|   IBIS model for TI AM261
[IBIS Ver]   5.1
[Disclaimer]   Please be aware that in the absence of a written agreement
|   Texas Instruments(TI) assumes no liability for:
|   (1) The accuracy of the IBIS models provided to your company,
|   however, the IBIS model is compliant to industry standard
|   IQ Level 2a.  Refer to IBIS Quality Section below for
|   for full details.
|   (2) The proper functioning of these Models in your design
|   or for any resulting applications
|   (3) Infringement of patents, copyrights or intellectual
|   property rights resulting from your use of these
|   models.
|   TI provides IBIS Models as a service to our customers and
|   therefore reserves the right to limit distribution of the
|   Models.  The information is subject to change without notice.
[File Name]  zej.ibs
[File Rev]   0.1
|   -Initial version
|   -Updated Package model
[Date]   10 October 2024
[Source]   Texas Instruments Incorporated
[Copyright]   Property of Texas Instruments Incorporated.
|   Unauthorized reproduction and/or distribution is strictly.
|   prohibited.
|   This product is protected under copyright law and trade
|   secret law as an unpublished work.
|   Created 2012,(C) Copyright 1999-2012,
|   Texas Instruments Incorporated., All Rights Reserved.
|   These commodities are under the U.S. Government
|   distribution license control. As such,they are not to be
|   re-exported without the prior approval of the U.S.
|   Department of Commerce.
[Notes]
   ADC pins are marked as NC
   USB pins are marked as NC
   Clock pins are marked as NC
   nReset pin marked as NC
|   Revision History
|   GERNERAL COMMENT: All IBIS Quality Notes below reflect latest release
|   and version of IBIS File
|   File passes ibischk6.0 with 0 errors and 35 warnings
|   Component AM261
[Component] AM261
[Manufacturer] TEXAS INSTRUMENTS
[Package Model] AM261_ZEJ
[Package]
|   typ   min   max
R_pkg   0.17037   0.058312   0.31733
L_pkg   2.972e-9   9.974e-10   4.815e-9
C_pkg   4.94e-13   3.685e-13   7.579e-13
[Pin]   Signal_name   model_name
E11   VDD   POWER
F12   VDD   POWER
H12   VDD   POWER
K12   VDD   POWER
M12   VDD   POWER
E5   VDD   POWER
E7   VDD   POWER
E9   VDD   POWER
G5   VDD   POWER
J5   VDD   POWER
L5   VDD   POWER
M6   VDD   POWER
N9   VDDA18_LDO   POWER
N6   VDDA18_OSC_PLL   POWER
N4   VDDA18_USB   POWER
M10   VDDA33   POWER
M8   VDDA33   POWER
M4   VDDA33_USB   POWER
D10   VDDAR2   POWER
G4   VDDAR3   POWER
D6   VDDS18   POWER
D12   VDDS18   POWER
G13   VDDS18   POWER
K13   VDDS18   POWER
K4   VDDS18   POWER
E4   VDDS18   POWER
N13   VDDS18   POWER
D9   VDDS18   POWER
P4   VDDS18_LDO   POWER
D4   VDDSHV_A   POWER
D7   VDDSHV_A   POWER
D11   VDDSHV_A   POWER
F13   VDDSHV_A   POWER
J13   VDDSHV_A   POWER
L4   VDDSHV_B   POWER
N12   VDDSHV_C   POWER
J4   VDDSHV_D   POWER
H4   VDDSHV_D   POWER
M13   VDDSHV_E   POWER
N5   VDDSHV_F   POWER
N8   VDD_TEMP   NC
P11   ADC0_AIN0   NC
N11   ADC0_AIN1   NC
R11   ADC0_AIN2   NC
P12   ADC0_AIN3   NC
T12   ADC0_AIN4   NC
R12   ADC0_AIN5   NC
T13   ADC0_AIN6   NC
R10   ADC1_AIN0   NC
N10   ADC1_AIN1   NC
P10   ADC1_AIN2   NC
P9   ADC1_AIN3   NC
T9   ADC1_AIN4   NC
R9   ADC1_AIN5   NC
R8   ADC1_AIN6   NC
R7   ADC2_AIN0   NC
P7   ADC2_AIN1   NC
P8   ADC2_AIN2   NC
P6   ADC2_AIN3   NC
R6   ADC2_AIN4   NC
N7   ADC2_AIN5   NC
T6   ADC2_AIN6   NC
R13   ADC_CAL0   NC
T10   ADC_VREFHI_G0   NC
T7   ADC_VREFHI_G1   NC
T11   ADC_VREFLO_G0   NC
T8   ADC_VREFLO_G1   NC
T4   ATESTV1   NC
T5   DAC_OUT   NC
P13   DAC_VREF0   NC
N3   GPIO0   bc1833dv40dcpbfbp18ll_rxll_ssdlv
M3   GPIO1   bc1833dv40dcpbfbp18ll_rxll_ssdlv
L2   GPIO2   bc1833dv40dcpbfbp18ll_rxll_ssdlv
M2   GPIO3   bc1833dv40dcpbfbp18ll_ssdlv
N1   GPIO4   bc1833dv40dcpbfbp18ll_ssdlv
L3   GPIO5   bc1833dv40dcpbfbp18ll_rxll_ssdlv
N2   GPIO6   bc1833dv40dcpbfbp18ll_rxll_ssdlv
J3   GPIO7   bc1833dv40dcpbfbp18ll_rxll_ssdlv
K1   GPIO8   bc1833dv40dcpbfbp18ll_rxll_ssdlv
K2   GPIO9   bc1833dv40dcpbfbp18ll_rxll_ssdlv
J2   GPIO10   bc1833dv40dcpbfbp18ll_rxll_ssdlv
B11   GPIO11   bc1833dv40dcpbfbp18ll_rxll_ssdlh
A12   GPIO12   bc1833dv40dcpbfbp18ll_ssdlh
A10   GPIO13   bc1833dv40dcpbfbp18ll_ssdlh
A11   GPIO14   bc1833dv40dcpbfbp18ll_rxll_ssdlh
B9   GPIO15   bc1833dv40dcpbfbp18ll_rxll_ssdlh
B10   GPIO16   bc1833dv40dcpbfbp18ll_rxll_ssdlh
A9   GPIO17   bc1833dv40dcpbfbp18ll_rxll_ssdlh
C11   GPIO18   bc1833dv40dcpbfbp18ll_rxll_ssdlh
C10   GPIO19   bc1833dv40dcpbfbp18ll_rxll_ssdlh
D8   GPIO20   bc1833dv40dcpbfbp18ll_rxll_ssdlh
B8   GPIO21   bc1833dv40dcpbfbp18ll_rxll_ssdlh
C9   GPIO22   bc1833dv40dcpbfbp18ll_rxll_ssdlh
B7   GPIO23   bc1833dv40dcpbfbp18ll_rxll_ssdlh
A8   GPIO24   bc1833dv40dcpbfbp18ll_rxll_ssdlh
C8   GPIO25   bc1833dv40dcpbfbp18ll_rxll_ssdlh
A7   GPIO26   bc1833dv40dcpbfbp18ll_rxll_ssdlh
A6   GPIO27   bc1833dv40dcpbfbp18ll_rxll_ssdlh
B6   GPIO28   bc1833dv40dcpbfbp18ll_rxll_ssdlh
P16   GPIO29   bc1833dv40dcpbfbp18ll_rxll_ssdlv_135u
M14   GPIO30   bc1833dv40dcpbfbp18ll_rxll_ssdlv_135u
P14   GPIO31   bc1833dv40dcpbfbp18ll_rxll_ssdlh
P15   GPIO32   bc1833dv40dcpbfbp18ll_rxll_ssdlh
R16   GPIO33   bc1833dv40dcpbfbp18ll_rxll_ssdlh
N14   GPIO34   bc1833dv40dcpbfbp18ll_rxll_ssdlv_135u
L15   GPIO35   bc1833dv40dcpbfbp18ll_rxll_ssdlv_135u
M16   GPIO36   bc1833dv40dcpbfbp18ll_rxll_ssdlv_135u
N15   GPIO37   bc1833dv40dcpbfbp18ll_rxll_ssdlv_135u
N16   GPIO38   bc1833dv40dcpbfbp18ll_rxll_ssdlv_135u
L13   GPIO39   bc1833dv40dcpbfbp18ll_rxll_ssdlv_135u
M15   GPIO40   bc1833dv40dcpbfbp18ll_rxll_ssdlv_135u
L16   GPIO41   bc1833dv40dcpbfbp18ll_rxll_ssdlv_135u
L14   GPIO42   bc1833dv40dcpbfbp18ll_rxll_ssdlv_135u
A4   GPIO43   bc1833dv40dcpbfbp18ll_rxll_ssdlh_135u
A5   GPIO44   bc1833dv40dcpbfbp18ll_rxll_ssdlh_135u
B4   GPIO45   bc1833dv40dcpbfbp18ll_rxll_ssdlh_135u
C5   GPIO46   bc1833dv40dcpbfbp18ll_rxll_ssdlh_135u
A3   GPIO47   bc1833dv40dcpbfbp18ll_rxll_ssdlh_135u
A2   GPIO48   bc1833dv40dcpbfbp18ll_rxll_ssdlh_135u
B2   GPIO49   bc1833dv40dcpbfbp18ll_rxll_ssdlh_135u
C4   GPIO50   bc1833dv40dcpbfbp18ll_rxll_ssdlv
B1   GPIO51   bc1833dv40dcpbfbp18ll_rxll_ssdlv
C1   GPIO52   bc1833dv40dcpbfbp18ll_rxll_ssdlv
C2   GPIO53   bc1833dv40dcpbfbp18ll_rxll_ssdlv
D3   GPIO54   bc1833dv40dcpbfbp18ll_rxll_ssdlv
E3   GPIO55   bc1833dv40dcpbfbp18ll_rxll_ssdlv
F4   GPIO56   bc1833dv40dcpbfbp18ll_rxll_ssdlv
D2   GPIO57   bc1833dv40dcpbfbp18ll_rxll_ssdlv
D1   GPIO58   bc1833dv40dcpbfbp18ll_rxll_ssdlv
E2   GPIO59   bc1833dv40dcpbfbp18ll_rxll_ssdlv
E1   GPIO60   bc1833dv40dcpbfbp18ll_rxll_ssdlv
F2   GPIO61   bc1833dv40dcpbfbp18ll_rxll_ssdlv
F3   GPIO62   bc1833dv40dcpbfbp18ll_rxll_ssdlv
G3   GPIO66   bc1833dv40dcpbfbp18ll_rxll_ssdlv
G2   GPIO67   bc1833dv40dcpbfbp18ll_rxll_ssdlv
H3   GPIO68   bc1833dv40dcpbfbp18ll_rxll_ssdlv
H2   GPIO69   bc1833dv40dcpbfbp18ll_rxll_ssdlv
G1   GPIO70   bc1833dv40dcpbfbp18ll_rxll_ssdlv
R14   GPIO71   bc1833dv40dcpbfbp18ll_rxll_ssdlh
T14   GPIO72   bc1833dv40dcpbfbp18ll_rxll_ssdlh
T15   GPIO73   bc1833dv40dcpbfbp18ll_rxll_ssdlh
R15   GPIO74   bc1833dv40dcpbfbp18ll_rxll_ssdlh
M1   GPIO75   bc1833dv40dcpbfbp18ll_rxll_ssdlv
L1   GPIO76   bc1833dv40dcpbfbp18ll_rxll_ssdlv
K15   GPIO85   bc1833dv40dcpbfbp18ll_rxll_ssdlv_135u
K16   GPIO86   bc1833dv40dcpbfbp18ll_rxll_ssdlv_135u
F14   GPIO87   bc1833dv40dcpbfbp18ll_rxll_ssdlv_135u
E15   GPIO88   bc1833dv40dcpbfbp18ll_rxll_ssdlv_135u
E16   GPIO89   bc1833dv40dcpbfbp18ll_rxll_ssdlv_135u
E14   GPIO90   bc1833dv40dcpbfbp18ll_rxll_ssdlv_135u
H15   GPIO91   bc1833dv40dcpbfbp18ll_rxll_ssdlv_135u
G15   GPIO92   bc1833dv40dcpbfbp18ll_rxll_ssdlv_135u
K14   GPIO93   bc1833dv40dcpbfbp18ll_rxll_ssdlv_135u
H14   GPIO94   bc1833dv40dcpbfbp18ll_rxll_ssdlv_135u
G16   GPIO95   bc1833dv40dcpbfbp18ll_rxll_ssdlv_135u
J14   GPIO96   bc1833dv40dcpbfbp18ll_rxll_ssdlv_135u
F16   GPIO97   bc1833dv40dcpbfbp18ll_rxll_ssdlv_135u
H16   GPIO98   bc1833dv40dcpbfbp18ll_rxll_ssdlv_135u
J15   GPIO99   bc1833dv40dcpbfbp18ll_rxll_ssdlv_135u
J16   GPIO100   bc1833dv40dcpbfbp18ll_rxll_ssdlv_135u
F15   GPIO101   bc1833dv40dcpbfbp18ll_rxll_ssdlv_135u
G14   GPIO102   bc1833dv40dcpbfbp18ll_rxll_ssdlv_135u
E13   GPIO107   bc1833dv40dcpbfbp18ll_rxll_ssdlv_135u
D15   GPIO108   bc1833dv40dcpbfbp18ll_rxll_ssdlv_135u
D14   GPIO109   bc1833dv40dcpbfbp18ll_rxll_ssdlv_135u
D16   GPIO110   bc1833dv40dcpbfbp18ll_rxll_ssdlv_135u
P3   GPIO121   bc1833dv40dcpbfbp18ll_rxll_ssdlh
C15   GPIO122   bc1833dv40dcpbfbp18ll_rxll_ssdlh
A15   GPIO123   bc1833dv40dcpbfbp18ll_rxll_ssdlh
C16   GPIO124   bc1833dv40dcpbfbp18ll_rxll_ssdlh
C14   GPIO125   bc1833dv40dcpbfbp18ll_rxll_ssdlh
B16   GPIO126   bc1833dv40dcpbfbp18ll_rxll_ssdlh
A14   GPIO127   bc1833dv40dcpbfbp18ll_rxll_ssdlh
B15   GPIO128   bc1833dv40dcpbfbp18ll_rxll_ssdlh
B14   GPIO129   bc1833dv40dcpbfbp18ll_rxll_ssdlh
D13   GPIO130   bc1833dv40dcpbfbp18ll_rxll_ssdlh
C13   GPIO131   bc1833dv40dcpbfbp18ll_rxll_ssdlh
C12   GPIO132   bc1833dv40dcpbfbp18ll_rxll_ssdlh
B13   GPIO133   bc1833dv40dcpbfbp18ll_rxll_ssdlh
B12   GPIO134   bi2c1833dvfzp18_ssdlh
A13   GPIO135   bi2c1833dvfzp18_ssdlh
H1   GPIO138   bc1833dv40dcpbfbp18ll_rxll_ssdlv
R1   GPIO139   NC
P1   GPIO140   NC
P2   PORZ   ihhv1833dvhyp18ll_ssdhv
B3   SAFETY_ERRORN   bc1833dv40dcpbfbp18ll_ssdlh_135u
C6   TCK   iq1833dvtckpbfbp18ll_ssdhh_135u
D5   TDI   bc1833dv40dcpbfbp18ll_ssdlh_135u
B5   TDO   bc1833dv40dcpbfbp18ll_ssdlh_135u
P5   TEMPCAL   NC
C7   TMS   bc1833dv40dcpbfbp18ll_ssdlh_135u
H13   VNWA   POWER
K3   VPP   POWER
R5   VSYS_MON   NC
C3   WARMRSTN   bc1833dv40dcpbfbp18ll_od_fs_cmphdl_ssdlv
T3   XTAL_XI   NC
T2   XTAL_XO   NC
A1   VSS   GND
A16   VSS   GND
F5   VSS   GND
E6   VSS   GND
E8   VSS   GND
E10   VSS   GND
E12   VSS   GND
G6   VSS   GND
F6   VSS   GND
G7   VSS   GND
F7   VSS   GND
G8   VSS   GND
F8   VSS   GND
G9   VSS   GND
F9   VSS   GND
G10   VSS   GND
F10   VSS   GND
G11   VSS   GND
F11   VSS   GND
H6   VSS   GND
H7   VSS   GND
H8   VSS   GND
H9   VSS   GND
H10   VSS   GND
H11   VSS   GND
K5   VSS   GND
K6   VSS   GND
J6   VSS   GND
K7   VSS   GND
J7   VSS   GND
K8   VSS   GND
J8   VSS   GND
K9   VSS   GND
J9   VSS   GND
K10   VSS   GND
J10   VSS   GND
K11   VSS   GND
J11   VSS   GND
L6   VSS   GND
L7   VSS   GND
L8   VSS   GND
L9   VSS   GND
L10   VSS   GND
L11   VSS   GND
M5   VSS   GND
M7   VSS   GND
G12   VSS   GND
H5   VSS   GND
J12   VSS   GND
L12   VSS   GND
R2   VSS   GND
T1   VSS   GND
R3   VSS   GND
R4   VSS   GND
T16   VSS   GND
M9   VSSA   GND
M11   VSSA   GND
|   BC1833DV40DCPBFBP18LL_SSDLH
[Model Selector] bc1833dv40dcpbfbp18ll_ssdlh
|SC1 IS A SLEW RATE CONTROL PIN
|5% SUPPLY VARIATION MODES WITH 1.8V NOM SUPPLY
BC40D_H_PUPDOFF_5P_SC1_1P8  Cell operated at 1.8(nom)
|BC40D_H_PUPDOFF_5P_SC1_1P8; BUFFER WITH WEAK PULUP/PULLDOWN OFF AT 5% SUPPLY
|VARIATION WITH SC1=1 MEANING SLOW MODE OF OPERATION
BC40D_H_PD_ON_5P_!SC1_1P8  Cell operated at 1.8(nom)
|BC40D_H_PD_ON_5P_!SC1_1P8; BUFFER WITH WEAK_PULLDOWN_ON AT 5% SUPPLY
|VARIATION WITH SC1=0 MEANING FAST MODE OF OPERATION
BC40D_H_PD_ON_5P_SC1_1P8  Cell operated at 1.8(nom)
|BC40D_H_PD_ON_5P_SC1_1P8; BUFFER WITH WEAK_PULLDOWN_ON AT 5% SUPPLY
|VARIATION WITH SC1=1 MEANING SLOW MODE OF OPERATION
BC40D_H_PU_ON_5P_!SC1_1P8  Cell operated at 1.8(nom)
|BC40D_H_PU_ON_5P_!SC1_1P8; BUFFER WITH WEAK_PULLUP_ON AT 5% SUPPLY
|VARIATION WITH SC1=0 MEANING FAST MODE OF OPERATION
BC40D_H_PUPDOFF_5P_!SC1_1P8  Cell operated at 1.8(nom)
|BC40D_H_PUPDOFF_5P_!SC1_1P8; BUFFER WITH WEAK PULUP/PULLDOWN OFF AT 5% SUPPLY
|VARIATION WITH SC1=0 MEANING FAST MODE OF OPERATION
BC40D_H_PU_ON_5P_SC1_1P8  Cell operated at 1.8(nom)
|BC40D_H_PU_ON_5P_SC1_1P8; BUFFER WITH WEAK_PULLUP_ON AT 5% SUPPLY
|VARIATION WITH SC1=1 MEANING SLOW MODE OF OPERATION
|5% SUPPLY VARIATION MODES WITH 3.3V NOM SUPPLY
BC40D_H_PUPDOFF_5P_SC1_3P3  Cell operated at 3.3(nom)
|BC40D_H_PUPDOFF_5P_SC1_3P3; BUFFER WITH WEAK PULUP/PULLDOWN OFF AT 5% SUPPLY
|VARIATION WITH SC1=1 MEANING SLOW MODE OF OPERATION
BC40D_H_PD_ON_5P_!SC1_3P3  Cell operated at 3.3(nom)
|BC40D_H_PD_ON_5P_!SC1_3P3; BUFFER WITH WEAK_PULLDOWN_ON AT 5% SUPPLY
|VARIATION WITH SC1=0 MEANING FAST MODE OF OPERATION
BC40D_H_PD_ON_5P_SC1_3P3  Cell operated at 3.3(nom)
|BC40D_H_PD_ON_5P_SC1_3P3; BUFFER WITH WEAK_PULLDOWN_ON AT 5% SUPPLY
|VARIATION WITH SC1=1 MEANING SLOW MODE OF OPERATION
BC40D_H_PU_ON_5P_!SC1_3P3  Cell operated at 3.3(nom)
|BC40D_H_PU_ON_5P_!SC1_3P3; BUFFER WITH WEAK_PULLUP_ON AT 5% SUPPLY
|VARIATION WITH SC1=0 MEANING FAST MODE OF OPERATION
BC40D_H_PUPDOFF_5P_!SC1_3P3  Cell operated at 3.3(nom)
|BC40D_H_PUPDOFF_5P_!SC1_3P3; BUFFER WITH WEAK PULUP/PULLDOWN OFF AT 5% SUPPLY
|VARIATION WITH SC1=0 MEANING FAST MODE OF OPERATION
BC40D_H_PU_ON_5P_SC1_3P3  Cell operated at 3.3(nom)
|BC40D_H_PU_ON_5P_SC1_3P3; BUFFER WITH WEAK_PULLUP_ON AT 5% SUPPLY
|VARIATION WITH SC1=1 MEANING SLOW MODE OF OPERATION
| 10% SUPPLY VARIATION MODES WITH 1.8V NOM SUPPLY
BC40D_H_PUPDOFF_10P_SC1_1P8  Cell operated at 1.8(nom)
|BC40D_H_PUPDOFF_10P_SC1_1P8; BUFFER WITH WEAK PULUP/PULLDOWN OFF AT 10% SUPPLY
|VARIATION WITH SC1=1 MEANING SLOW MODE OF OPERATION
BC40D_H_PD_ON_10P_!SC1_1P8  Cell operated at 1.8(nom)
|BC40D_H_PD_ON_10P_!SC1_1P8; BUFFER WITH WEAK_PULLDOWN_ON AT 10% SUPPLY
|VARIATION WITH SC1=0 MEANING FAST MODE OF OPERATION
BC40D_H_PD_ON_10P_SC1_1P8  Cell operated at 1.8(nom)
|BC40D_H_PD_ON_10P_SC1_1P8; BUFFER WITH WEAK_PULLDOWN_ON AT 10% SUPPLY
|VARIATION WITH SC1=1 MEANING SLOW MODE OF OPERATION
BC40D_H_PU_ON_10P_!SC1_1P8  Cell operated at 1.8(nom)
|BC40D_H_PU_ON_10P_!SC1_1P8; BUFFER WITH WEAK_PULLUP_ON AT 10% SUPPLY
|VARIATION WITH SC1=0 MEANING FAST MODE OF OPERATION
BC40D_H_PUPDOFF_10P_!SC1_1P8  Cell operated at 1.8(nom)
|BC40D_H_PUPDOFF_10P_!SC1_1P8; BUFFER WITH WEAK PULUP/PULLDOWN OFF AT 10% SUPPLY
|VARIATION WITH SC1=0 MEANING FAST MODE OF OPERATION
BC40D_H_PU_ON_10P_SC1_1P8  Cell operated at 1.8(nom)
|BC40D_H_PU_ON_10P_SC1_1P8; BUFFER WITH WEAK_PULLUP_ON AT 10% SUPPLY
|VARIATION WITH SC1=1 MEANING SLOW MODE OF OPERATION
| 10% SUPPLY VARIATION MODES WITH 3.3V NOM SUPPLY
BC40D_H_PUPDOFF_10P_SC1_3P3  Cell operated at 3.3(nom)
|BC40D_H_PUPDOFF_10P_SC1_3P3; BUFFER WITH WEAK PULUP/PULLDOWN OFF AT 10% SUPPLY
|VARIATION WITH SC1=1 MEANING SLOW MODE OF OPERATION
BC40D_H_PD_ON_10P_!SC1_3P3  Cell operated at 3.3(nom)
|BC40D_H_PD_ON_10P_!SC1_3P3; BUFFER WITH WEAK_PULLDOWN_ON 10% SUPPLY
|VARIATION WITH SC1=0 MEANING FAST MODE OF OPERATION
BC40D_H_PD_ON_10P_SC1_3P3  Cell operated at 3.3(nom)
|BC40D_H_PD_ON_10P_SC1_3P3; BUFFER WITH WEAK_PULLDOWN_ON AT 10% SUPPLY
|VARIATION WITH SC1=1 MEANING SLOW MODE OF OPERATION
BC40D_H_PU_ON_10P_!SC1_3P3  Cell operated at 3.3(nom)
|BC40D_H_PU_ON_10P_!SC1_3P3; BUFFER WITH WEAK_PULLUP_ON AT 10% SUPPLY
|VARIATION WITH SC1=0 MEANING FAST MODE OF OPERATION
BC40D_H_PUPDOFF_10P_!SC1_3P3  Cell operated at 3.3(nom)
|BC40D_H_PUPDOFF_10P_!SC1_3P3; BUFFER WITH WEAK PULUP/PULLDOWN OFF AT 10% SUPPLY
|VARIATION WITH SC1=0 MEANING FAST MODE OF OPERATION
BC40D_H_PU_ON_10P_SC1_3P3  Cell operated at 3.3(nom)
|BC40D_H_PU_ON_10P_SC1_3P3; BUFFER WITH WEAK_PULLUP_ON AT 10% SUPPLY
|VARIATION WITH SC1=1 MEANING SLOW MODE OF OPERATION
|   BC1833DV40DCPBFBP18LL_SSDLV
[Model Selector] bc1833dv40dcpbfbp18ll_ssdlv
|SC1 IS A SLEW RATE CONTROL PIN
|5% SUPPLY VARIATION MODES WITH 1.8V NOM SUPPLY
BC40D_V_PUPDOFF_5P_SC1_1P8  Cell operated at 1.8(nom)
|BC40D_V_PUPDOFF_5P_SC1_1P8; BUFFER WITH WEAK PULUP/PULLDOWN OFF AT 5% SUPPLY
|VARIATION WITH SC1=1 MEANING SLOW MODE OF OPERATION
BC40D_V_PD_ON_5P_!SC1_1P8  Cell operated at 1.8(nom)
|BC40D_V_PD_ON_5P_!SC1_1P8; BUFFER WITH WEAK_PULLDOWN_ON AT 5% SUPPLY
|VARIATION WITH SC1=0 MEANING FAST MODE OF OPERATION
BC40D_V_PD_ON_5P_SC1_1P8  Cell operated at 1.8(nom)
|BC40D_V_PD_ON_5P_SC1_1P8; BUFFER WITH WEAK_PULLDOWN_ON AT 5% SUPPLY
|VARIATION WITH SC1=1 MEANING SLOW MODE OF OPERATION
BC40D_V_PU_ON_5P_!SC1_1P8  Cell operated at 1.8(nom)
|BC40D_V_PU_ON_5P_!SC1_1P8; BUFFER WITH WEAK_PULLUP_ON AT 5% SUPPLY
|VARIATION WITH SC1=0 MEANING FAST MODE OF OPERATION
BC40D_V_PUPDOFF_5P_!SC1_1P8  Cell operated at 1.8(nom)
|BC40D_V_PUPDOFF_5P_!SC1_1P8; BUFFER WITH WEAK PULUP/PULLDOWN OFF AT 5% SUPPLY
|VARIATION WITH SC1=0 MEANING FAST MODE OF OPERATION
BC40D_V_PU_ON_5P_SC1_1P8  Cell operated at 1.8(nom)
|BC40D_V_PU_ON_5P_SC1_1P8; BUFFER WITH WEAK_PULLUP_ON AT 5% SUPPLY
|VARIATION WITH SC1=1 MEANING SLOW MODE OF OPERATION
|5% SUPPLY VARIATION MODES WITH 3.3V NOM SUPPLY
BC40D_V_PUPDOFF_5P_SC1_3P3  Cell operated at 3.3(nom)
|BC40D_V_PUPDOFF_5P_SC1_3P3; BUFFER WITH WEAK PULUP/PULLDOWN OFF AT 5% SUPPLY
|VARIATION WITH SC1=1 MEANING SLOW MODE OF OPERATION
BC40D_V_PD_ON_5P_!SC1_3P3  Cell operated at 3.3(nom)
|BC40D_V_PD_ON_5P_!SC1_3P3; BUFFER WITH WEAK_PULLDOWN_ON AT 5% SUPPLY
|VARIATION WITH SC1=0 MEANING FAST MODE OF OPERATION
BC40D_V_PD_ON_5P_SC1_3P3  Cell operated at 3.3(nom)
|BC40D_V_PD_ON_5P_SC1_3P3; BUFFER WITH WEAK_PULLDOWN_ON AT 5% SUPPLY
|VARIATION WITH SC1=1 MEANING SLOW MODE OF OPERATION
BC40D_V_PU_ON_5P_!SC1_3P3  Cell operated at 3.3(nom)
|BC40D_V_PU_ON_5P_!SC1_3P3; BUFFER WITH WEAK_PULLUP_ON AT 5% SUPPLY
|VARIATION WITH SC1=0 MEANING FAST MODE OF OPERATION
BC40D_V_PUPDOFF_5P_!SC1_3P3  Cell operated at 3.3(nom)
|BC40D_V_PUPDOFF_5P_!SC1_3P3; BUFFER WITH WEAK PULUP/PULLDOWN OFF AT 5% SUPPLY
|VARIATION WITH SC1=0 MEANING FAST MODE OF OPERATION
BC40D_V_PU_ON_5P_SC1_3P3  Cell operated at 3.3(nom)
|BC40D_V_PU_ON_5P_SC1_3P3; BUFFER WITH WEAK_PULLUP_ON AT 5% SUPPLY
|VARIATION WITH SC1=1 MEANING SLOW MODE OF OPERATION
| 10% SUPPLY VARIATION MODES WITH 1.8V NOM SUPPLY
BC40D_V_PUPDOFF_10P_SC1_1P8  Cell operated at 1.8(nom)
|BC40D_V_PUPDOFF_10P_SC1_1P8; BUFFER WITH WEAK PULUP/PULLDOWN OFF AT 10% SUPPLY
|VARIATION WITH SC1=1 MEANING SLOW MODE OF OPERATION
BC40D_V_PD_ON_10P_!SC1_1P8  Cell operated at 1.8(nom)
|BC40D_V_PD_ON_10P_!SC1_1P8; BUFFER WITH WEAK_PULLDOWN_ON AT 10% SUPPLY
|VARIATION WITH SC1=0 MEANING FAST MODE OF OPERATION
BC40D_V_PD_ON_10P_SC1_1P8  Cell operated at 1.8(nom)
|BC40D_V_PD_ON_10P_SC1_1P8; BUFFER WITH WEAK_PULLDOWN_ON AT 10% SUPPLY
|VARIATION WITH SC1=1 MEANING SLOW MODE OF OPERATION
BC40D_V_PU_ON_10P_!SC1_1P8  Cell operated at 1.8(nom)
|BC40D_V_PU_ON_10P_!SC1_1P8; BUFFER WITH WEAK_PULLUP_ON AT 10% SUPPLY
|VARIATION WITH SC1=0 MEANING FAST MODE OF OPERATION
BC40D_V_PUPDOFF_10P_!SC1_1P8  Cell operated at 1.8(nom)
|BC40D_V_PUPDOFF_10P_!SC1_1P8; BUFFER WITH WEAK PULUP/PULLDOWN OFF AT 10% SUPPLY
|VARIATION WITH SC1=0 MEANING FAST MODE OF OPERATION
BC40D_V_PU_ON_10P_SC1_1P8  Cell operated at 1.8(nom)
|BC40D_V_PU_ON_10P_SC1_1P8; BUFFER WITH WEAK_PULLUP_ON AT 10% SUPPLY
|VARIATION WITH SC1=1 MEANING SLOW MODE OF OPERATION
| 10% SUPPLY VARIATION MODES WITH 3.3V NOM SUPPLY
BC40D_V_PUPDOFF_10P_SC1_3P3  Cell operated at 3.3(nom)
|BC40D_V_PUPDOFF_10P_SC1_3P3; BUFFER WITH WEAK PULUP/PULLDOWN OFF AT 10% SUPPLY
|VARIATION WITH SC1=1 MEANING SLOW MODE OF OPERATION
BC40D_V_PD_ON_10P_!SC1_3P3  Cell operated at 3.3(nom)
|BC40D_V_PD_ON_10P_!SC1_3P3; BUFFER WITH WEAK_PULLDOWN_ON 10% SUPPLY
|VARIATION WITH SC1=0 MEANING FAST MODE OF OPERATION
BC40D_V_PD_ON_10P_SC1_3P3  Cell operated at 3.3(nom)
|BC40D_V_PD_ON_10P_SC1_3P3; BUFFER WITH WEAK_PULLDOWN_ON AT 10% SUPPLY
|VARIATION WITH SC1=1 MEANING SLOW MODE OF OPERATION
BC40D_V_PU_ON_10P_!SC1_3P3  Cell operated at 3.3(nom)
|BC40D_V_PU_ON_10P_!SC1_3P3; BUFFER WITH WEAK_PULLUP_ON AT 10% SUPPLY
|VARIATION WITH SC1=0 MEANING FAST MODE OF OPERATION
BC40D_V_PUPDOFF_10P_!SC1_3P3  Cell operated at 3.3(nom)
|BC40D_V_PUPDOFF_10P_!SC1_3P3; BUFFER WITH WEAK PULUP/PULLDOWN OFF AT 10% SUPPLY
|VARIATION WITH SC1=0 MEANING FAST MODE OF OPERATION
BC40D_V_PU_ON_10P_SC1_3P3  Cell operated at 3.3(nom)
|BC40D_V_PU_ON_10P_SC1_3P3; BUFFER WITH WEAK_PULLUP_ON AT 10% SUPPLY
|VARIATION WITH SC1=1 MEANING SLOW MODE OF OPERATION
|   BI2C1833DVFZP18_SSDLH
[Model Selector] bi2c1833dvfzp18_ssdlh
BI2C1833_NORAML_5P_1P8  Cell operated at 1.8(nom)
|BI2C1833_NORAML_5P_1P8; I2C MODE AT 1.8V WITH 5% SUPPLY VARIATION
BI2C1833_NORAML_5P_3P3  Cell operated at 3.3(nom)
|BI2C1833_NORAML_5P_3P3; I2C MODE AT 3.3V WITH 5% SUPPLY VARIATION
BI2C1833_NORAML_10P_1P8  Cell operated at 1.8(nom)
|BI2C1833_NORAML_10P_1P8; I2C MODE AT 1.8V WITH 10% SUPPLY VARIATION
BI2C1833_NORAML_10P_3P3  Cell operated at 3.3(nom)
|BI2C1833_NORAML_10P_3P3; I2C MODE AT 3.3V WITH 10% SUPPLY VARIATION
|   IHHV1833DVHYP18LL_SSDHV
[Model Selector] ihhv1833dvhyp18ll_ssdhv
IHHV_NORAML_5P_1P8  Cell operated at 1.8(nom)
|IHHV_NORAML_5P_1P8; NORMAL MODE AT 1.8V WITH 5% SUPPLY VARIATION
IHHV_NORAML_5P_3P3  Cell operated at 3.3(nom)
|IHHV_NORAML_5P_3P3; NORMAL MODE AT 3.3V WITH 5% SUPPLY VARIATION
IHHV_NORAML_10P_1P8  Cell operated at 1.8(nom)
|IHHV_NORAML_10P_1P8; NORMAL MODE AT 1.8V WITH 10% SUPPLY VARIATION
IHHV_NORAML_10P_3P3  Cell operated at 3.3(nom)
|IHHV_NORAML_10P_3P3; NORMAL MODE AT 3.3V WITH 10% SUPPLY VARIATION
|   BC1833DV40DCPBFBP18LL_OD_FS_CMPHDL_SSDLV
[Model Selector] bc1833dv40dcpbfbp18ll_od_fs_cmphdl_ssdlv
|SC1 IS A SLEW RATE CONTROL PIN
|5% SUPPLY VARIATION MODES WITH 1.8V NOM SUPPLY
BC40D_V_PUPDOFF_5P_SC1_1P8  Cell operated at 1.8(nom)
|BC40D_V_PUPDOFF_5P_SC1_1P8; BUFFER WITH WEAK PULUP/PULLDOWN OFF AT 5% SUPPLY
|VARIATION WITH SC1=1 MEANING SLOW MODE OF OPERATION
BC40D_V_PD_ON_5P_!SC1_1P8  Cell operated at 1.8(nom)
|BC40D_V_PD_ON_5P_!SC1_1P8; BUFFER WITH WEAK_PULLDOWN_ON AT 5% SUPPLY
|VARIATION WITH SC1=0 MEANING FAST MODE OF OPERATION
BC40D_V_PD_ON_5P_SC1_1P8  Cell operated at 1.8(nom)
|BC40D_V_PD_ON_5P_SC1_1P8; BUFFER WITH WEAK_PULLDOWN_ON AT 5% SUPPLY
|VARIATION WITH SC1=1 MEANING SLOW MODE OF OPERATION
BC40D_V_PU_ON_5P_!SC1_1P8  Cell operated at 1.8(nom)
|BC40D_V_PU_ON_5P_!SC1_1P8; BUFFER WITH WEAK_PULLUP_ON AT 5% SUPPLY
|VARIATION WITH SC1=0 MEANING FAST MODE OF OPERATION
BC40D_V_PUPDOFF_5P_!SC1_1P8  Cell operated at 1.8(nom)
|BC40D_V_PUPDOFF_5P_!SC1_1P8; BUFFER WITH WEAK PULUP/PULLDOWN OFF AT 5% SUPPLY
|VARIATION WITH SC1=0 MEANING FAST MODE OF OPERATION
BC40D_V_PU_ON_5P_SC1_1P8  Cell operated at 1.8(nom)
|BC40D_V_PU_ON_5P_SC1_1P8; BUFFER WITH WEAK_PULLUP_ON AT 5% SUPPLY
|VARIATION WITH SC1=1 MEANING SLOW MODE OF OPERATION
|5% SUPPLY VARIATION MODES WITH 3.3V NOM SUPPLY
BC40D_V_PUPDOFF_5P_SC1_3P3  Cell operated at 3.3(nom)
|BC40D_V_PUPDOFF_5P_SC1_3P3; BUFFER WITH WEAK PULUP/PULLDOWN OFF AT 5% SUPPLY
|VARIATION WITH SC1=1 MEANING SLOW MODE OF OPERATION
BC40D_V_PD_ON_5P_!SC1_3P3  Cell operated at 3.3(nom)
|BC40D_V_PD_ON_5P_!SC1_3P3; BUFFER WITH WEAK_PULLDOWN_ON AT 5% SUPPLY
|VARIATION WITH SC1=0 MEANING FAST MODE OF OPERATION
BC40D_V_PD_ON_5P_SC1_3P3  Cell operated at 3.3(nom)
|BC40D_V_PD_ON_5P_SC1_3P3; BUFFER WITH WEAK_PULLDOWN_ON AT 5% SUPPLY
|VARIATION WITH SC1=1 MEANING SLOW MODE OF OPERATION
BC40D_V_PU_ON_5P_!SC1_3P3  Cell operated at 3.3(nom)
|BC40D_V_PU_ON_5P_!SC1_3P3; BUFFER WITH WEAK_PULLUP_ON AT 5% SUPPLY
|VARIATION WITH SC1=0 MEANING FAST MODE OF OPERATION
BC40D_V_PUPDOFF_5P_!SC1_3P3  Cell operated at 3.3(nom)
|BC40D_V_PUPDOFF_5P_!SC1_3P3; BUFFER WITH WEAK PULUP/PULLDOWN OFF AT 5% SUPPLY
|VARIATION WITH SC1=0 MEANING FAST MODE OF OPERATION
BC40D_V_PU_ON_5P_SC1_3P3  Cell operated at 3.3(nom)
|BC40D_V_PU_ON_5P_SC1_3P3; BUFFER WITH WEAK_PULLUP_ON AT 5% SUPPLY
|VARIATION WITH SC1=1 MEANING SLOW MODE OF OPERATION
| 10% SUPPLY VARIATION MODES WITH 1.8V NOM SUPPLY
BC40D_V_PUPDOFF_10P_SC1_1P8  Cell operated at 1.8(nom)
|BC40D_V_PUPDOFF_10P_SC1_1P8; BUFFER WITH WEAK PULUP/PULLDOWN OFF AT 10% SUPPLY
|VARIATION WITH SC1=1 MEANING SLOW MODE OF OPERATION
BC40D_V_PD_ON_10P_!SC1_1P8  Cell operated at 1.8(nom)
|BC40D_V_PD_ON_10P_!SC1_1P8; BUFFER WITH WEAK_PULLDOWN_ON AT 10% SUPPLY
|VARIATION WITH SC1=0 MEANING FAST MODE OF OPERATION
BC40D_V_PD_ON_10P_SC1_1P8  Cell operated at 1.8(nom)
|BC40D_V_PD_ON_10P_SC1_1P8; BUFFER WITH WEAK_PULLDOWN_ON AT 10% SUPPLY
|VARIATION WITH SC1=1 MEANING SLOW MODE OF OPERATION
BC40D_V_PU_ON_10P_!SC1_1P8  Cell operated at 1.8(nom)
|BC40D_V_PU_ON_10P_!SC1_1P8; BUFFER WITH WEAK_PULLUP_ON AT 10% SUPPLY
|VARIATION WITH SC1=0 MEANING FAST MODE OF OPERATION
BC40D_V_PUPDOFF_10P_!SC1_1P8  Cell operated at 1.8(nom)
|BC40D_V_PUPDOFF_10P_!SC1_1P8; BUFFER WITH WEAK PULUP/PULLDOWN OFF AT 10% SUPPLY
|VARIATION WITH SC1=0 MEANING FAST MODE OF OPERATION
BC40D_V_PU_ON_10P_SC1_1P8  Cell operated at 1.8(nom)
|BC40D_V_PU_ON_10P_SC1_1P8; BUFFER WITH WEAK_PULLUP_ON AT 10% SUPPLY
|VARIATION WITH SC1=1 MEANING SLOW MODE OF OPERATION
| 10% SUPPLY VARIATION MODES WITH 3.3V NOM SUPPLY
BC40D_V_PUPDOFF_10P_SC1_3P3  Cell operated at 3.3(nom)
|BC40D_V_PUPDOFF_10P_SC1_3P3; BUFFER WITH WEAK PULUP/PULLDOWN OFF AT 10% SUPPLY
|VARIATION WITH SC1=1 MEANING SLOW MODE OF OPERATION
BC40D_V_PD_ON_10P_!SC1_3P3  Cell operated at 3.3(nom)
|BC40D_V_PD_ON_10P_!SC1_3P3; BUFFER WITH WEAK_PULLDOWN_ON 10% SUPPLY
|VARIATION WITH SC1=0 MEANING FAST MODE OF OPERATION
BC40D_V_PD_ON_10P_SC1_3P3  Cell operated at 3.3(nom)
|BC40D_V_PD_ON_10P_SC1_3P3; BUFFER WITH WEAK_PULLDOWN_ON AT 10% SUPPLY
|VARIATION WITH SC1=1 MEANING SLOW MODE OF OPERATION
BC40D_V_PU_ON_10P_!SC1_3P3  Cell operated at 3.3(nom)
|BC40D_V_PU_ON_10P_!SC1_3P3; BUFFER WITH WEAK_PULLUP_ON AT 10% SUPPLY
|VARIATION WITH SC1=0 MEANING FAST MODE OF OPERATION
BC40D_V_PUPDOFF_10P_!SC1_3P3  Cell operated at 3.3(nom)
|BC40D_V_PUPDOFF_10P_!SC1_3P3; BUFFER WITH WEAK PULUP/PULLDOWN OFF AT 10% SUPPLY
|VARIATION WITH SC1=0 MEANING FAST MODE OF OPERATION
BC40D_V_PU_ON_10P_SC1_3P3  Cell operated at 3.3(nom)
|BC40D_V_PU_ON_10P_SC1_3P3; BUFFER WITH WEAK_PULLUP_ON AT 10% SUPPLY
|VARIATION WITH SC1=1 MEANING SLOW MODE OF OPERATION
|   IQ1833DVTCKPBFBP18LL_SSDHH_135U
[Model Selector] iq1833dvtckpbfbp18ll_ssdhh_135u
|5% SUPPLY VARIATION MODES WITH 1.8V NOM SUPPLY
IQ_SSDHH_PD_ON_5P_1P8  Cell operated at 1.8(nom)
|IQ_SSDHH_PD_ON_5P_1P8; BUFFER WITH WEAK_PULLDOWN_ON AT 5% SUPPLY VARIATION
IQ_SSDHH_PU_ON_5P_1P8  Cell operated at 1.8(nom)
|IQ_SSDHH_PU_ON_5P_1P8; BUFFER WITH WEAK_PULLUP_ON AT 5% SUPPLY VARIATION
IQ_SSDHH_PUPDOFF_5P_1P8  Cell operated at 1.8(nom)
|IQ_SSDHH_PUPDOFF_5P_1P8; BUFFER WITH WEAK PUPD OFF AT 5% SUPPLY VARIATION
|5% SUPPLY VARIATION MODES WITH 3.3V NOM SUPPLY
IQ_SSDHH_PD_ON_5P_3P3  Cell operated at 3.3(nom)
|IQ_SSDHH_PD_ON_5P_3P3; BUFFER WITH WEAK_PULLDOWN_ON AT 5% SUPPLY VARIATION
IQ_SSDHH_PU_ON_5P_3P3  Cell operated at 3.3(nom)
|IQ_SSDHH_PU_ON_5P_3P3; BUFFER WITH WEAK_PULLUP_ON AT 5% SUPPLY VARIATION
IQ_SSDHH_PUPDOFF_5P_3P3  Cell operated at 3.3(nom)
|IQ_SSDHH_PUPDOFF_5P_3P3; BUFFER WITH WEAK PUPD OFF AT 5% SUPPLY VARIATION
|10% SUPPLY VARIATION MODES WITH 1.8V NOM SUPPLY
IQ_SSDHH_PD_ON_10P_1P8  Cell operated at 1.8(nom)
|IQ_SSDHH_PD_ON_10P_1P8; BUFFER WITH WEAK_PULLDOWN_ON AT 10% SUPPLY VARIATION
IQ_SSDHH_PU_ON_10P_1P8  Cell operated at 1.8(nom)
|IQ_SSDHH_PU_ON_10P_1P8; BUFFER WITH WEAK_PULLUP_ON AT 10% SUPPLY VARIATION
IQ_SSDHH_PUPDOFF_10P_1P8  Cell operated at 1.8(nom)
|IQ_SSDHH_PUPDOFF_10P_1P8; BUFFER WITH WEAK PUPD OFF AT 10% SUPPLY VARIATION
|10% SUPPLY VARIATION MODES WITH 3.3V NOM SUPPLY
IQ_SSDHH_PD_ON_10P_3P3  Cell operated at 3.3(nom)
|IQ_SSDHH_PD_ON_10P_3P3; BUFFER WITH WEAK_PULLDOWN_ON  AT 10% SUPPLY VARIATION
IQ_SSDHH_PU_ON_10P_3P3  Cell operated at 3.3(nom)
|IQ_SSDHH_PU_ON_10P_3P3; BUFFER WITH WEAK_PULLUP_ON AT 10% SUPPLY VARIATION
IQ_SSDHH_PUPDOFF_10P_3P3  Cell operated at 3.3(nom)
|IQ_SSDHH_PUPDOFF_10P_3P3; BUFFER WITH WEAK PUPD OFF AT 10% SUPPLY VARIATION
|   BC1833DV40DCPBFBP18LL_RXLL_SSDLH
[Model Selector] bc1833dv40dcpbfbp18ll_rxll_ssdlh
|SC1 IS A SLEW RATE CONTROL PIN
|5% SUPPLY VARIATION MODES WITH 1.8V NOM SUPPLY
BC40D_H_PUPDOFF_5P_SC1_1P8  Cell operated at 1.8(nom)
|BC40D_H_PUPDOFF_5P_SC1_1P8; BUFFER WITH WEAK PULUP/PULLDOWN OFF AT 5% SUPPLY
|VARIATION WITH SC1=1 MEANING SLOW MODE OF OPERATION
BC40D_H_PD_ON_5P_!SC1_1P8  Cell operated at 1.8(nom)
|BC40D_H_PD_ON_5P_!SC1_1P8; BUFFER WITH WEAK_PULLDOWN_ON AT 5% SUPPLY
|VARIATION WITH SC1=0 MEANING FAST MODE OF OPERATION
BC40D_H_PD_ON_5P_SC1_1P8  Cell operated at 1.8(nom)
|BC40D_H_PD_ON_5P_SC1_1P8; BUFFER WITH WEAK_PULLDOWN_ON AT 5% SUPPLY
|VARIATION WITH SC1=1 MEANING SLOW MODE OF OPERATION
BC40D_H_PU_ON_5P_!SC1_1P8  Cell operated at 1.8(nom)
|BC40D_H_PU_ON_5P_!SC1_1P8; BUFFER WITH WEAK_PULLUP_ON AT 5% SUPPLY
|VARIATION WITH SC1=0 MEANING FAST MODE OF OPERATION
BC40D_H_PUPDOFF_5P_!SC1_1P8  Cell operated at 1.8(nom)
|BC40D_H_PUPDOFF_5P_!SC1_1P8; BUFFER WITH WEAK PULUP/PULLDOWN OFF AT 5% SUPPLY
|VARIATION WITH SC1=0 MEANING FAST MODE OF OPERATION
BC40D_H_PU_ON_5P_SC1_1P8  Cell operated at 1.8(nom)
|BC40D_H_PU_ON_5P_SC1_1P8; BUFFER WITH WEAK_PULLUP_ON AT 5% SUPPLY
|VARIATION WITH SC1=1 MEANING SLOW MODE OF OPERATION
|5% SUPPLY VARIATION MODES WITH 3.3V NOM SUPPLY
BC40D_H_PUPDOFF_5P_SC1_3P3  Cell operated at 3.3(nom)
|BC40D_H_PUPDOFF_5P_SC1_3P3; BUFFER WITH WEAK PULUP/PULLDOWN OFF AT 5% SUPPLY
|VARIATION WITH SC1=1 MEANING SLOW MODE OF OPERATION
BC40D_H_PD_ON_5P_!SC1_3P3  Cell operated at 3.3(nom)
|BC40D_H_PD_ON_5P_!SC1_3P3; BUFFER WITH WEAK_PULLDOWN_ON AT 5% SUPPLY
|VARIATION WITH SC1=0 MEANING FAST MODE OF OPERATION
BC40D_H_PD_ON_5P_SC1_3P3  Cell operated at 3.3(nom)
|BC40D_H_PD_ON_5P_SC1_3P3; BUFFER WITH WEAK_PULLDOWN_ON AT 5% SUPPLY
|VARIATION WITH SC1=1 MEANING SLOW MODE OF OPERATION
BC40D_H_PU_ON_5P_!SC1_3P3  Cell operated at 3.3(nom)
|BC40D_H_PU_ON_5P_!SC1_3P3; BUFFER WITH WEAK_PULLUP_ON AT 5% SUPPLY
|VARIATION WITH SC1=0 MEANING FAST MODE OF OPERATION
BC40D_H_PUPDOFF_5P_!SC1_3P3  Cell operated at 3.3(nom)
|BC40D_H_PUPDOFF_5P_!SC1_3P3; BUFFER WITH WEAK PULUP/PULLDOWN OFF AT 5% SUPPLY
|VARIATION WITH SC1=0 MEANING FAST MODE OF OPERATION
BC40D_H_PU_ON_5P_SC1_3P3  Cell operated at 3.3(nom)
|BC40D_H_PU_ON_5P_SC1_3P3; BUFFER WITH WEAK_PULLUP_ON AT 5% SUPPLY
|VARIATION WITH SC1=1 MEANING SLOW MODE OF OPERATION
| 10% SUPPLY VARIATION MODES WITH 1.8V NOM SUPPLY
BC40D_H_PUPDOFF_10P_SC1_1P8  Cell operated at 1.8(nom)
|BC40D_H_PUPDOFF_10P_SC1_1P8; BUFFER WITH WEAK PULUP/PULLDOWN OFF AT 10% SUPPLY
|VARIATION WITH SC1=1 MEANING SLOW MODE OF OPERATION
BC40D_H_PD_ON_10P_!SC1_1P8  Cell operated at 1.8(nom)
|BC40D_H_PD_ON_10P_!SC1_1P8; BUFFER WITH WEAK_PULLDOWN_ON AT 10% SUPPLY
|VARIATION WITH SC1=0 MEANING FAST MODE OF OPERATION
BC40D_H_PD_ON_10P_SC1_1P8  Cell operated at 1.8(nom)
|BC40D_H_PD_ON_10P_SC1_1P8; BUFFER WITH WEAK_PULLDOWN_ON AT 10% SUPPLY
|VARIATION WITH SC1=1 MEANING SLOW MODE OF OPERATION
BC40D_H_PU_ON_10P_!SC1_1P8  Cell operated at 1.8(nom)
|BC40D_H_PU_ON_10P_!SC1_1P8; BUFFER WITH WEAK_PULLUP_ON AT 10% SUPPLY
|VARIATION WITH SC1=0 MEANING FAST MODE OF OPERATION
BC40D_H_PUPDOFF_10P_!SC1_1P8  Cell operated at 1.8(nom)
|BC40D_H_PUPDOFF_10P_!SC1_1P8; BUFFER WITH WEAK PULUP/PULLDOWN OFF AT 10% SUPPLY
|VARIATION WITH SC1=0 MEANING FAST MODE OF OPERATION
BC40D_H_PU_ON_10P_SC1_1P8  Cell operated at 1.8(nom)
|BC40D_H_PU_ON_10P_SC1_1P8; BUFFER WITH WEAK_PULLUP_ON AT 10% SUPPLY
|VARIATION WITH SC1=1 MEANING SLOW MODE OF OPERATION
| 10% SUPPLY VARIATION MODES WITH 3.3V NOM SUPPLY
BC40D_H_PUPDOFF_10P_SC1_3P3  Cell operated at 3.3(nom)
|BC40D_H_PUPDOFF_10P_SC1_3P3; BUFFER WITH WEAK PULUP/PULLDOWN OFF AT 10% SUPPLY
|VARIATION WITH SC1=1 MEANING SLOW MODE OF OPERATION
BC40D_H_PD_ON_10P_!SC1_3P3  Cell operated at 3.3(nom)
|BC40D_H_PD_ON_10P_!SC1_3P3; BUFFER WITH WEAK_PULLDOWN_ON 10% SUPPLY
|VARIATION WITH SC1=0 MEANING FAST MODE OF OPERATION
BC40D_H_PD_ON_10P_SC1_3P3  Cell operated at 3.3(nom)
|BC40D_H_PD_ON_10P_SC1_3P3; BUFFER WITH WEAK_PULLDOWN_ON AT 10% SUPPLY
|VARIATION WITH SC1=1 MEANING SLOW MODE OF OPERATION
BC40D_H_PU_ON_10P_!SC1_3P3  Cell operated at 3.3(nom)
|BC40D_H_PU_ON_10P_!SC1_3P3; BUFFER WITH WEAK_PULLUP_ON AT 10% SUPPLY
|VARIATION WITH SC1=0 MEANING FAST MODE OF OPERATION
BC40D_H_PUPDOFF_10P_!SC1_3P3  Cell operated at 3.3(nom)
|BC40D_H_PUPDOFF_10P_!SC1_3P3; BUFFER WITH WEAK PULUP/PULLDOWN OFF AT 10% SUPPLY
|VARIATION WITH SC1=0 MEANING FAST MODE OF OPERATION
BC40D_H_PU_ON_10P_SC1_3P3  Cell operated at 3.3(nom)
|BC40D_H_PU_ON_10P_SC1_3P3; BUFFER WITH WEAK_PULLUP_ON AT 10% SUPPLY
|VARIATION WITH SC1=1 MEANING SLOW MODE OF OPERATION
|   BC1833DV40DCPBFBP18LL_RXLL_SSDLV
[Model Selector] bc1833dv40dcpbfbp18ll_rxll_ssdlv
|SC1 IS A SLEW RATE CONTROL PIN
|5% SUPPLY VARIATION MODES WITH 1.8V NOM SUPPLY
BC40D_V_PUPDOFF_5P_SC1_1P8  Cell operated at 1.8(nom)
|BC40D_V_PUPDOFF_5P_SC1_1P8; BUFFER WITH WEAK PULUP/PULLDOWN OFF AT 5% SUPPLY
|VARIATION WITH SC1=1 MEANING SLOW MODE OF OPERATION
BC40D_V_PD_ON_5P_!SC1_1P8  Cell operated at 1.8(nom)
|BC40D_V_PD_ON_5P_!SC1_1P8; BUFFER WITH WEAK_PULLDOWN_ON AT 5% SUPPLY
|VARIATION WITH SC1=0 MEANING FAST MODE OF OPERATION
BC40D_V_PD_ON_5P_SC1_1P8  Cell operated at 1.8(nom)
|BC40D_V_PD_ON_5P_SC1_1P8; BUFFER WITH WEAK_PULLDOWN_ON AT 5% SUPPLY
|VARIATION WITH SC1=1 MEANING SLOW MODE OF OPERATION
BC40D_V_PU_ON_5P_!SC1_1P8  Cell operated at 1.8(nom)
|BC40D_V_PU_ON_5P_!SC1_1P8; BUFFER WITH WEAK_PULLUP_ON AT 5% SUPPLY
|VARIATION WITH SC1=0 MEANING FAST MODE OF OPERATION
BC40D_V_PUPDOFF_5P_!SC1_1P8  Cell operated at 1.8(nom)
|BC40D_V_PUPDOFF_5P_!SC1_1P8; BUFFER WITH WEAK PULUP/PULLDOWN OFF AT 5% SUPPLY
|VARIATION WITH SC1=0 MEANING FAST MODE OF OPERATION
BC40D_V_PU_ON_5P_SC1_1P8  Cell operated at 1.8(nom)
|BC40D_V_PU_ON_5P_SC1_1P8; BUFFER WITH WEAK_PULLUP_ON AT 5% SUPPLY
|VARIATION WITH SC1=1 MEANING SLOW MODE OF OPERATION
|5% SUPPLY VARIATION MODES WITH 3.3V NOM SUPPLY
BC40D_V_PUPDOFF_5P_SC1_3P3  Cell operated at 3.3(nom)
|BC40D_V_PUPDOFF_5P_SC1_3P3; BUFFER WITH WEAK PULUP/PULLDOWN OFF AT 5% SUPPLY
|VARIATION WITH SC1=1 MEANING SLOW MODE OF OPERATION
BC40D_V_PD_ON_5P_!SC1_3P3  Cell operated at 3.3(nom)
|BC40D_V_PD_ON_5P_!SC1_3P3; BUFFER WITH WEAK_PULLDOWN_ON AT 5% SUPPLY
|VARIATION WITH SC1=0 MEANING FAST MODE OF OPERATION
BC40D_V_PD_ON_5P_SC1_3P3  Cell operated at 3.3(nom)
|BC40D_V_PD_ON_5P_SC1_3P3; BUFFER WITH WEAK_PULLDOWN_ON AT 5% SUPPLY
|VARIATION WITH SC1=1 MEANING SLOW MODE OF OPERATION
BC40D_V_PU_ON_5P_!SC1_3P3  Cell operated at 3.3(nom)
|BC40D_V_PU_ON_5P_!SC1_3P3; BUFFER WITH WEAK_PULLUP_ON AT 5% SUPPLY
|VARIATION WITH SC1=0 MEANING FAST MODE OF OPERATION
BC40D_V_PUPDOFF_5P_!SC1_3P3  Cell operated at 3.3(nom)
|BC40D_V_PUPDOFF_5P_!SC1_3P3; BUFFER WITH WEAK PULUP/PULLDOWN OFF AT 5% SUPPLY
|VARIATION WITH SC1=0 MEANING FAST MODE OF OPERATION
BC40D_V_PU_ON_5P_SC1_3P3  Cell operated at 3.3(nom)
|BC40D_V_PU_ON_5P_SC1_3P3; BUFFER WITH WEAK_PULLUP_ON AT 5% SUPPLY
|VARIATION WITH SC1=1 MEANING SLOW MODE OF OPERATION
| 10% SUPPLY VARIATION MODES WITH 1.8V NOM SUPPLY
BC40D_V_PUPDOFF_10P_SC1_1P8  Cell operated at 1.8(nom)
|BC40D_V_PUPDOFF_10P_SC1_1P8; BUFFER WITH WEAK PULUP/PULLDOWN OFF AT 10% SUPPLY
|VARIATION WITH SC1=1 MEANING SLOW MODE OF OPERATION
BC40D_V_PD_ON_10P_!SC1_1P8  Cell operated at 1.8(nom)
|BC40D_V_PD_ON_10P_!SC1_1P8; BUFFER WITH WEAK_PULLDOWN_ON AT 10% SUPPLY
|VARIATION WITH SC1=0 MEANING FAST MODE OF OPERATION
BC40D_V_PD_ON_10P_SC1_1P8  Cell operated at 1.8(nom)
|BC40D_V_PD_ON_10P_SC1_1P8; BUFFER WITH WEAK_PULLDOWN_ON AT 10% SUPPLY
|VARIATION WITH SC1=1 MEANING SLOW MODE OF OPERATION
BC40D_V_PU_ON_10P_!SC1_1P8  Cell operated at 1.8(nom)
|BC40D_V_PU_ON_10P_!SC1_1P8; BUFFER WITH WEAK_PULLUP_ON AT 10% SUPPLY
|VARIATION WITH SC1=0 MEANING FAST MODE OF OPERATION
BC40D_V_PUPDOFF_10P_!SC1_1P8  Cell operated at 1.8(nom)
|BC40D_V_PUPDOFF_10P_!SC1_1P8; BUFFER WITH WEAK PULUP/PULLDOWN OFF AT 10% SUPPLY
|VARIATION WITH SC1=0 MEANING FAST MODE OF OPERATION
BC40D_V_PU_ON_10P_SC1_1P8  Cell operated at 1.8(nom)
|BC40D_V_PU_ON_10P_SC1_1P8; BUFFER WITH WEAK_PULLUP_ON AT 10% SUPPLY
|VARIATION WITH SC1=1 MEANING SLOW MODE OF OPERATION
| 10% SUPPLY VARIATION MODES WITH 3.3V NOM SUPPLY
BC40D_V_PUPDOFF_10P_SC1_3P3  Cell operated at 3.3(nom)
|BC40D_V_PUPDOFF_10P_SC1_3P3; BUFFER WITH WEAK PULUP/PULLDOWN OFF AT 10% SUPPLY
|VARIATION WITH SC1=1 MEANING SLOW MODE OF OPERATION
BC40D_V_PD_ON_10P_!SC1_3P3  Cell operated at 3.3(nom)
|BC40D_V_PD_ON_10P_!SC1_3P3; BUFFER WITH WEAK_PULLDOWN_ON 10% SUPPLY
|VARIATION WITH SC1=0 MEANING FAST MODE OF OPERATION
BC40D_V_PD_ON_10P_SC1_3P3  Cell operated at 3.3(nom)
|BC40D_V_PD_ON_10P_SC1_3P3; BUFFER WITH WEAK_PULLDOWN_ON AT 10% SUPPLY
|VARIATION WITH SC1=1 MEANING SLOW MODE OF OPERATION
BC40D_V_PU_ON_10P_!SC1_3P3  Cell operated at 3.3(nom)
|BC40D_V_PU_ON_10P_!SC1_3P3; BUFFER WITH WEAK_PULLUP_ON AT 10% SUPPLY
|VARIATION WITH SC1=0 MEANING FAST MODE OF OPERATION
BC40D_V_PUPDOFF_10P_!SC1_3P3  Cell operated at 3.3(nom)
|BC40D_V_PUPDOFF_10P_!SC1_3P3; BUFFER WITH WEAK PULUP/PULLDOWN OFF AT 10% SUPPLY
|VARIATION WITH SC1=0 MEANING FAST MODE OF OPERATION
BC40D_V_PU_ON_10P_SC1_3P3  Cell operated at 3.3(nom)
|BC40D_V_PU_ON_10P_SC1_3P3; BUFFER WITH WEAK_PULLUP_ON AT 10% SUPPLY
|VARIATION WITH SC1=1 MEANING SLOW MODE OF OPERATION
|   BC1833DV40DCPBFBP18LL_RXLL_SSDLH_135U
[Model Selector] bc1833dv40dcpbfbp18ll_rxll_ssdlh_135u
|SC1 IS A SLEW RATE CONTROL PIN
|5% SUPPLY VARIATION MODES WITH 1.8V NOM SUPPLY
BC40D_H_PUPDOFF_5P_SC1_1P8  Cell operated at 1.8(nom)
|BC40D_H_PUPDOFF_5P_SC1_1P8; BUFFER WITH WEAK PULUP/PULLDOWN OFF AT 5% SUPPLY
|VARIATION WITH SC1=1 MEANING SLOW MODE OF OPERATION
BC40D_H_PD_ON_5P_!SC1_1P8  Cell operated at 1.8(nom)
|BC40D_H_PD_ON_5P_!SC1_1P8; BUFFER WITH WEAK_PULLDOWN_ON AT 5% SUPPLY
|VARIATION WITH SC1=0 MEANING FAST MODE OF OPERATION
BC40D_H_PD_ON_5P_SC1_1P8  Cell operated at 1.8(nom)
|BC40D_H_PD_ON_5P_SC1_1P8; BUFFER WITH WEAK_PULLDOWN_ON AT 5% SUPPLY
|VARIATION WITH SC1=1 MEANING SLOW MODE OF OPERATION
BC40D_H_PU_ON_5P_!SC1_1P8  Cell operated at 1.8(nom)
|BC40D_H_PU_ON_5P_!SC1_1P8; BUFFER WITH WEAK_PULLUP_ON AT 5% SUPPLY
|VARIATION WITH SC1=0 MEANING FAST MODE OF OPERATION
BC40D_H_PUPDOFF_5P_!SC1_1P8  Cell operated at 1.8(nom)
|BC40D_H_PUPDOFF_5P_!SC1_1P8; BUFFER WITH WEAK PULUP/PULLDOWN OFF AT 5% SUPPLY
|VARIATION WITH SC1=0 MEANING FAST MODE OF OPERATION
BC40D_H_PU_ON_5P_SC1_1P8  Cell operated at 1.8(nom)
|BC40D_H_PU_ON_5P_SC1_1P8; BUFFER WITH WEAK_PULLUP_ON AT 5% SUPPLY
|VARIATION WITH SC1=1 MEANING SLOW MODE OF OPERATION
|5% SUPPLY VARIATION MODES WITH 3.3V NOM SUPPLY
BC40D_H_PUPDOFF_5P_SC1_3P3  Cell operated at 3.3(nom)
|BC40D_H_PUPDOFF_5P_SC1_3P3; BUFFER WITH WEAK PULUP/PULLDOWN OFF AT 5% SUPPLY
|VARIATION WITH SC1=1 MEANING SLOW MODE OF OPERATION
BC40D_H_PD_ON_5P_!SC1_3P3  Cell operated at 3.3(nom)
|BC40D_H_PD_ON_5P_!SC1_3P3; BUFFER WITH WEAK_PULLDOWN_ON AT 5% SUPPLY
|VARIATION WITH SC1=0 MEANING FAST MODE OF OPERATION
BC40D_H_PD_ON_5P_SC1_3P3  Cell operated at 3.3(nom)
|BC40D_H_PD_ON_5P_SC1_3P3; BUFFER WITH WEAK_PULLDOWN_ON AT 5% SUPPLY
|VARIATION WITH SC1=1 MEANING SLOW MODE OF OPERATION
BC40D_H_PU_ON_5P_!SC1_3P3  Cell operated at 3.3(nom)
|BC40D_H_PU_ON_5P_!SC1_3P3; BUFFER WITH WEAK_PULLUP_ON AT 5% SUPPLY
|VARIATION WITH SC1=0 MEANING FAST MODE OF OPERATION
BC40D_H_PUPDOFF_5P_!SC1_3P3  Cell operated at 3.3(nom)
|BC40D_H_PUPDOFF_5P_!SC1_3P3; BUFFER WITH WEAK PULUP/PULLDOWN OFF AT 5% SUPPLY
|VARIATION WITH SC1=0 MEANING FAST MODE OF OPERATION
BC40D_H_PU_ON_5P_SC1_3P3  Cell operated at 3.3(nom)
|BC40D_H_PU_ON_5P_SC1_3P3; BUFFER WITH WEAK_PULLUP_ON AT 5% SUPPLY
|VARIATION WITH SC1=1 MEANING SLOW MODE OF OPERATION
| 10% SUPPLY VARIATION MODES WITH 1.8V NOM SUPPLY
BC40D_H_PUPDOFF_10P_SC1_1P8  Cell operated at 1.8(nom)
|BC40D_H_PUPDOFF_10P_SC1_1P8; BUFFER WITH WEAK PULUP/PULLDOWN OFF AT 10% SUPPLY
|VARIATION WITH SC1=1 MEANING SLOW MODE OF OPERATION
BC40D_H_PD_ON_10P_!SC1_1P8  Cell operated at 1.8(nom)
|BC40D_H_PD_ON_10P_!SC1_1P8; BUFFER WITH WEAK_PULLDOWN_ON AT 10% SUPPLY
|VARIATION WITH SC1=0 MEANING FAST MODE OF OPERATION
BC40D_H_PD_ON_10P_SC1_1P8  Cell operated at 1.8(nom)
|BC40D_H_PD_ON_10P_SC1_1P8; BUFFER WITH WEAK_PULLDOWN_ON AT 10% SUPPLY
|VARIATION WITH SC1=1 MEANING SLOW MODE OF OPERATION
BC40D_H_PU_ON_10P_!SC1_1P8  Cell operated at 1.8(nom)
|BC40D_H_PU_ON_10P_!SC1_1P8; BUFFER WITH WEAK_PULLUP_ON AT 10% SUPPLY
|VARIATION WITH SC1=0 MEANING FAST MODE OF OPERATION
BC40D_H_PUPDOFF_10P_!SC1_1P8  Cell operated at 1.8(nom)
|BC40D_H_PUPDOFF_10P_!SC1_1P8; BUFFER WITH WEAK PULUP/PULLDOWN OFF AT 10% SUPPLY
|VARIATION WITH SC1=0 MEANING FAST MODE OF OPERATION
BC40D_H_PU_ON_10P_SC1_1P8  Cell operated at 1.8(nom)
|BC40D_H_PU_ON_10P_SC1_1P8; BUFFER WITH WEAK_PULLUP_ON AT 10% SUPPLY
|VARIATION WITH SC1=1 MEANING SLOW MODE OF OPERATION
| 10% SUPPLY VARIATION MODES WITH 3.3V NOM SUPPLY
BC40D_H_PUPDOFF_10P_SC1_3P3  Cell operated at 3.3(nom)
|BC40D_H_PUPDOFF_10P_SC1_3P3; BUFFER WITH WEAK PULUP/PULLDOWN OFF AT 10% SUPPLY
|VARIATION WITH SC1=1 MEANING SLOW MODE OF OPERATION
BC40D_H_PD_ON_10P_!SC1_3P3  Cell operated at 3.3(nom)
|BC40D_H_PD_ON_10P_!SC1_3P3; BUFFER WITH WEAK_PULLDOWN_ON 10% SUPPLY
|VARIATION WITH SC1=0 MEANING FAST MODE OF OPERATION
BC40D_H_PD_ON_10P_SC1_3P3  Cell operated at 3.3(nom)
|BC40D_H_PD_ON_10P_SC1_3P3; BUFFER WITH WEAK_PULLDOWN_ON AT 10% SUPPLY
|VARIATION WITH SC1=1 MEANING SLOW MODE OF OPERATION
BC40D_H_PU_ON_10P_!SC1_3P3  Cell operated at 3.3(nom)
|BC40D_H_PU_ON_10P_!SC1_3P3; BUFFER WITH WEAK_PULLUP_ON AT 10% SUPPLY
|VARIATION WITH SC1=0 MEANING FAST MODE OF OPERATION
BC40D_H_PUPDOFF_10P_!SC1_3P3  Cell operated at 3.3(nom)
|BC40D_H_PUPDOFF_10P_!SC1_3P3; BUFFER WITH WEAK PULUP/PULLDOWN OFF AT 10% SUPPLY
|VARIATION WITH SC1=0 MEANING FAST MODE OF OPERATION
BC40D_H_PU_ON_10P_SC1_3P3  Cell operated at 3.3(nom)
|BC40D_H_PU_ON_10P_SC1_3P3; BUFFER WITH WEAK_PULLUP_ON AT 10% SUPPLY
|VARIATION WITH SC1=1 MEANING SLOW MODE OF OPERATION
|   BC1833DV40DCPBFBP18LL_RXLL_SSDLV_135U
[Model Selector] bc1833dv40dcpbfbp18ll_rxll_ssdlv_135u
|SC1 IS A SLEW RATE CONTROL PIN
|5% SUPPLY VARIATION MODES WITH 1.8V NOM SUPPLY
BC40D_V_PUPDOFF_5P_SC1_1P8  Cell operated at 1.8(nom)
|BC40D_V_PUPDOFF_5P_SC1_1P8; BUFFER WITH WEAK PULUP/PULLDOWN OFF AT 5% SUPPLY
|VARIATION WITH SC1=1 MEANING SLOW MODE OF OPERATION
BC40D_V_PD_ON_5P_!SC1_1P8  Cell operated at 1.8(nom)
|BC40D_V_PD_ON_5P_!SC1_1P8; BUFFER WITH WEAK_PULLDOWN_ON AT 5% SUPPLY
|VARIATION WITH SC1=0 MEANING FAST MODE OF OPERATION
BC40D_V_PD_ON_5P_SC1_1P8  Cell operated at 1.8(nom)
|BC40D_V_PD_ON_5P_SC1_1P8; BUFFER WITH WEAK_PULLDOWN_ON AT 5% SUPPLY
|VARIATION WITH SC1=1 MEANING SLOW MODE OF OPERATION
BC40D_V_PU_ON_5P_!SC1_1P8  Cell operated at 1.8(nom)
|BC40D_V_PU_ON_5P_!SC1_1P8; BUFFER WITH WEAK_PULLUP_ON AT 5% SUPPLY
|VARIATION WITH SC1=0 MEANING FAST MODE OF OPERATION
BC40D_V_PUPDOFF_5P_!SC1_1P8  Cell operated at 1.8(nom)
|BC40D_V_PUPDOFF_5P_!SC1_1P8; BUFFER WITH WEAK PULUP/PULLDOWN OFF AT 5% SUPPLY
|VARIATION WITH SC1=0 MEANING FAST MODE OF OPERATION
BC40D_V_PU_ON_5P_SC1_1P8  Cell operated at 1.8(nom)
|BC40D_V_PU_ON_5P_SC1_1P8; BUFFER WITH WEAK_PULLUP_ON AT 5% SUPPLY
|VARIATION WITH SC1=1 MEANING SLOW MODE OF OPERATION
|5% SUPPLY VARIATION MODES WITH 3.3V NOM SUPPLY
BC40D_V_PUPDOFF_5P_SC1_3P3  Cell operated at 3.3(nom)
|BC40D_V_PUPDOFF_5P_SC1_3P3; BUFFER WITH WEAK PULUP/PULLDOWN OFF AT 5% SUPPLY
|VARIATION WITH SC1=1 MEANING SLOW MODE OF OPERATION
BC40D_V_PD_ON_5P_!SC1_3P3  Cell operated at 3.3(nom)
|BC40D_V_PD_ON_5P_!SC1_3P3; BUFFER WITH WEAK_PULLDOWN_ON AT 5% SUPPLY
|VARIATION WITH SC1=0 MEANING FAST MODE OF OPERATION
BC40D_V_PD_ON_5P_SC1_3P3  Cell operated at 3.3(nom)
|BC40D_V_PD_ON_5P_SC1_3P3; BUFFER WITH WEAK_PULLDOWN_ON AT 5% SUPPLY
|VARIATION WITH SC1=1 MEANING SLOW MODE OF OPERATION
BC40D_V_PU_ON_5P_!SC1_3P3  Cell operated at 3.3(nom)
|BC40D_V_PU_ON_5P_!SC1_3P3; BUFFER WITH WEAK_PULLUP_ON AT 5% SUPPLY
|VARIATION WITH SC1=0 MEANING FAST MODE OF OPERATION
BC40D_V_PUPDOFF_5P_!SC1_3P3  Cell operated at 3.3(nom)
|BC40D_V_PUPDOFF_5P_!SC1_3P3; BUFFER WITH WEAK PULUP/PULLDOWN OFF AT 5% SUPPLY
|VARIATION WITH SC1=0 MEANING FAST MODE OF OPERATION
BC40D_V_PU_ON_5P_SC1_3P3  Cell operated at 3.3(nom)
|BC40D_V_PU_ON_5P_SC1_3P3; BUFFER WITH WEAK_PULLUP_ON AT 5% SUPPLY
|VARIATION WITH SC1=1 MEANING SLOW MODE OF OPERATION
| 10% SUPPLY VARIATION MODES WITH 1.8V NOM SUPPLY
BC40D_V_PUPDOFF_10P_SC1_1P8  Cell operated at 1.8(nom)
|BC40D_V_PUPDOFF_10P_SC1_1P8; BUFFER WITH WEAK PULUP/PULLDOWN OFF AT 10% SUPPLY
|VARIATION WITH SC1=1 MEANING SLOW MODE OF OPERATION
BC40D_V_PD_ON_10P_!SC1_1P8  Cell operated at 1.8(nom)
|BC40D_V_PD_ON_10P_!SC1_1P8; BUFFER WITH WEAK_PULLDOWN_ON AT 10% SUPPLY
|VARIATION WITH SC1=0 MEANING FAST MODE OF OPERATION
BC40D_V_PD_ON_10P_SC1_1P8  Cell operated at 1.8(nom)
|BC40D_V_PD_ON_10P_SC1_1P8; BUFFER WITH WEAK_PULLDOWN_ON AT 10% SUPPLY
|VARIATION WITH SC1=1 MEANING SLOW MODE OF OPERATION
BC40D_V_PU_ON_10P_!SC1_1P8  Cell operated at 1.8(nom)
|BC40D_V_PU_ON_10P_!SC1_1P8; BUFFER WITH WEAK_PULLUP_ON AT 10% SUPPLY
|VARIATION WITH SC1=0 MEANING FAST MODE OF OPERATION
BC40D_V_PUPDOFF_10P_!SC1_1P8  Cell operated at 1.8(nom)
|BC40D_V_PUPDOFF_10P_!SC1_1P8; BUFFER WITH WEAK PULUP/PULLDOWN OFF AT 10% SUPPLY
|VARIATION WITH SC1=0 MEANING FAST MODE OF OPERATION
BC40D_V_PU_ON_10P_SC1_1P8  Cell operated at 1.8(nom)
|BC40D_V_PU_ON_10P_SC1_1P8; BUFFER WITH WEAK_PULLUP_ON AT 10% SUPPLY
|VARIATION WITH SC1=1 MEANING SLOW MODE OF OPERATION
| 10% SUPPLY VARIATION MODES WITH 3.3V NOM SUPPLY
BC40D_V_PUPDOFF_10P_SC1_3P3  Cell operated at 3.3(nom)
|BC40D_V_PUPDOFF_10P_SC1_3P3; BUFFER WITH WEAK PULUP/PULLDOWN OFF AT 10% SUPPLY
|VARIATION WITH SC1=1 MEANING SLOW MODE OF OPERATION
BC40D_V_PD_ON_10P_!SC1_3P3  Cell operated at 3.3(nom)
|BC40D_V_PD_ON_10P_!SC1_3P3; BUFFER WITH WEAK_PULLDOWN_ON 10% SUPPLY
|VARIATION WITH SC1=0 MEANING FAST MODE OF OPERATION
BC40D_V_PD_ON_10P_SC1_3P3  Cell operated at 3.3(nom)
|BC40D_V_PD_ON_10P_SC1_3P3; BUFFER WITH WEAK_PULLDOWN_ON AT 10% SUPPLY
|VARIATION WITH SC1=1 MEANING SLOW MODE OF OPERATION
BC40D_V_PU_ON_10P_!SC1_3P3  Cell operated at 3.3(nom)
|BC40D_V_PU_ON_10P_!SC1_3P3; BUFFER WITH WEAK_PULLUP_ON AT 10% SUPPLY
|VARIATION WITH SC1=0 MEANING FAST MODE OF OPERATION
BC40D_V_PUPDOFF_10P_!SC1_3P3  Cell operated at 3.3(nom)
|BC40D_V_PUPDOFF_10P_!SC1_3P3; BUFFER WITH WEAK PULUP/PULLDOWN OFF AT 10% SUPPLY
|VARIATION WITH SC1=0 MEANING FAST MODE OF OPERATION
BC40D_V_PU_ON_10P_SC1_3P3  Cell operated at 3.3(nom)
|BC40D_V_PU_ON_10P_SC1_3P3; BUFFER WITH WEAK_PULLUP_ON AT 10% SUPPLY
|VARIATION WITH SC1=1 MEANING SLOW MODE OF OPERATION
|   BC1833DV40DCPBFBP18LL_SSDLH_135U
[Model Selector] bc1833dv40dcpbfbp18ll_ssdlh_135u
|SC1 IS A SLEW RATE CONTROL PIN
|5% SUPPLY VARIATION MODES WITH 1.8V NOM SUPPLY
BC40D_H_PUPDOFF_5P_SC1_1P8  Cell operated at 1.8(nom)
|BC40D_H_PUPDOFF_5P_SC1_1P8; BUFFER WITH WEAK PULUP/PULLDOWN OFF AT 5% SUPPLY
|VARIATION WITH SC1=1 MEANING SLOW MODE OF OPERATION
BC40D_H_PD_ON_5P_!SC1_1P8  Cell operated at 1.8(nom)
|BC40D_H_PD_ON_5P_!SC1_1P8; BUFFER WITH WEAK_PULLDOWN_ON AT 5% SUPPLY
|VARIATION WITH SC1=0 MEANING FAST MODE OF OPERATION
BC40D_H_PD_ON_5P_SC1_1P8  Cell operated at 1.8(nom)
|BC40D_H_PD_ON_5P_SC1_1P8; BUFFER WITH WEAK_PULLDOWN_ON AT 5% SUPPLY
|VARIATION WITH SC1=1 MEANING SLOW MODE OF OPERATION
BC40D_H_PU_ON_5P_!SC1_1P8  Cell operated at 1.8(nom)
|BC40D_H_PU_ON_5P_!SC1_1P8; BUFFER WITH WEAK_PULLUP_ON AT 5% SUPPLY
|VARIATION WITH SC1=0 MEANING FAST MODE OF OPERATION
BC40D_H_PUPDOFF_5P_!SC1_1P8  Cell operated at 1.8(nom)
|BC40D_H_PUPDOFF_5P_!SC1_1P8; BUFFER WITH WEAK PULUP/PULLDOWN OFF AT 5% SUPPLY
|VARIATION WITH SC1=0 MEANING FAST MODE OF OPERATION
BC40D_H_PU_ON_5P_SC1_1P8  Cell operated at 1.8(nom)
|BC40D_H_PU_ON_5P_SC1_1P8; BUFFER WITH WEAK_PULLUP_ON AT 5% SUPPLY
|VARIATION WITH SC1=1 MEANING SLOW MODE OF OPERATION
|5% SUPPLY VARIATION MODES WITH 3.3V NOM SUPPLY
BC40D_H_PUPDOFF_5P_SC1_3P3  Cell operated at 3.3(nom)
|BC40D_H_PUPDOFF_5P_SC1_3P3; BUFFER WITH WEAK PULUP/PULLDOWN OFF AT 5% SUPPLY
|VARIATION WITH SC1=1 MEANING SLOW MODE OF OPERATION
BC40D_H_PD_ON_5P_!SC1_3P3  Cell operated at 3.3(nom)
|BC40D_H_PD_ON_5P_!SC1_3P3; BUFFER WITH WEAK_PULLDOWN_ON AT 5% SUPPLY
|VARIATION WITH SC1=0 MEANING FAST MODE OF OPERATION
BC40D_H_PD_ON_5P_SC1_3P3  Cell operated at 3.3(nom)
|BC40D_H_PD_ON_5P_SC1_3P3; BUFFER WITH WEAK_PULLDOWN_ON AT 5% SUPPLY
|VARIATION WITH SC1=1 MEANING SLOW MODE OF OPERATION
BC40D_H_PU_ON_5P_!SC1_3P3  Cell operated at 3.3(nom)
|BC40D_H_PU_ON_5P_!SC1_3P3; BUFFER WITH WEAK_PULLUP_ON AT 5% SUPPLY
|VARIATION WITH SC1=0 MEANING FAST MODE OF OPERATION
BC40D_H_PUPDOFF_5P_!SC1_3P3  Cell operated at 3.3(nom)
|BC40D_H_PUPDOFF_5P_!SC1_3P3; BUFFER WITH WEAK PULUP/PULLDOWN OFF AT 5% SUPPLY
|VARIATION WITH SC1=0 MEANING FAST MODE OF OPERATION
BC40D_H_PU_ON_5P_SC1_3P3  Cell operated at 3.3(nom)
|BC40D_H_PU_ON_5P_SC1_3P3; BUFFER WITH WEAK_PULLUP_ON AT 5% SUPPLY
|VARIATION WITH SC1=1 MEANING SLOW MODE OF OPERATION
| 10% SUPPLY VARIATION MODES WITH 1.8V NOM SUPPLY
BC40D_H_PUPDOFF_10P_SC1_1P8  Cell operated at 1.8(nom)
|BC40D_H_PUPDOFF_10P_SC1_1P8; BUFFER WITH WEAK PULUP/PULLDOWN OFF AT 10% SUPPLY
|VARIATION WITH SC1=1 MEANING SLOW MODE OF OPERATION
BC40D_H_PD_ON_10P_!SC1_1P8  Cell operated at 1.8(nom)
|BC40D_H_PD_ON_10P_!SC1_1P8; BUFFER WITH WEAK_PULLDOWN_ON AT 10% SUPPLY
|VARIATION WITH SC1=0 MEANING FAST MODE OF OPERATION
BC40D_H_PD_ON_10P_SC1_1P8  Cell operated at 1.8(nom)
|BC40D_H_PD_ON_10P_SC1_1P8; BUFFER WITH WEAK_PULLDOWN_ON AT 10% SUPPLY
|VARIATION WITH SC1=1 MEANING SLOW MODE OF OPERATION
BC40D_H_PU_ON_10P_!SC1_1P8  Cell operated at 1.8(nom)
|BC40D_H_PU_ON_10P_!SC1_1P8; BUFFER WITH WEAK_PULLUP_ON AT 10% SUPPLY
|VARIATION WITH SC1=0 MEANING FAST MODE OF OPERATION
BC40D_H_PUPDOFF_10P_!SC1_1P8  Cell operated at 1.8(nom)
|BC40D_H_PUPDOFF_10P_!SC1_1P8; BUFFER WITH WEAK PULUP/PULLDOWN OFF AT 10% SUPPLY
|VARIATION WITH SC1=0 MEANING FAST MODE OF OPERATION
BC40D_H_PU_ON_10P_SC1_1P8  Cell operated at 1.8(nom)
|BC40D_H_PU_ON_10P_SC1_1P8; BUFFER WITH WEAK_PULLUP_ON AT 10% SUPPLY
|VARIATION WITH SC1=1 MEANING SLOW MODE OF OPERATION
| 10% SUPPLY VARIATION MODES WITH 3.3V NOM SUPPLY
BC40D_H_PUPDOFF_10P_SC1_3P3  Cell operated at 3.3(nom)
|BC40D_H_PUPDOFF_10P_SC1_3P3; BUFFER WITH WEAK PULUP/PULLDOWN OFF AT 10% SUPPLY
|VARIATION WITH SC1=1 MEANING SLOW MODE OF OPERATION
BC40D_H_PD_ON_10P_!SC1_3P3  Cell operated at 3.3(nom)
|BC40D_H_PD_ON_10P_!SC1_3P3; BUFFER WITH WEAK_PULLDOWN_ON 10% SUPPLY
|VARIATION WITH SC1=0 MEANING FAST MODE OF OPERATION
BC40D_H_PD_ON_10P_SC1_3P3  Cell operated at 3.3(nom)
|BC40D_H_PD_ON_10P_SC1_3P3; BUFFER WITH WEAK_PULLDOWN_ON AT 10% SUPPLY
|VARIATION WITH SC1=1 MEANING SLOW MODE OF OPERATION
BC40D_H_PU_ON_10P_!SC1_3P3  Cell operated at 3.3(nom)
|BC40D_H_PU_ON_10P_!SC1_3P3; BUFFER WITH WEAK_PULLUP_ON AT 10% SUPPLY
|VARIATION WITH SC1=0 MEANING FAST MODE OF OPERATION
BC40D_H_PUPDOFF_10P_!SC1_3P3  Cell operated at 3.3(nom)
|BC40D_H_PUPDOFF_10P_!SC1_3P3; BUFFER WITH WEAK PULUP/PULLDOWN OFF AT 10% SUPPLY
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| Models and submodels in the file (68): BC40D_H_PUPDOFF_5P_SC1_1P8 (I/O), BC40D_H_PD_ON_5P_!SC1_1P8 (I/O), BC40D_H_PD_ON_5P_SC1_1P8 (I/O), BC40D_H_PU_ON_5P_!SC1_1P8 (I/O), BC40D_H_PUPDOFF_5P_!SC1_1P8 (I/O), BC40D_H_PU_ON_5P_SC1_1P8 (I/O), BC40D_H_PUPDOFF_5P_SC1_3P3 (I/O), BC40D_H_PD_ON_5P_!SC1_3P3 (I/O), BC40D_H_PD_ON_5P_SC1_3P3 (I/O), BC40D_H_PU_ON_5P_!SC1_3P3 (I/O), BC40D_H_PUPDOFF_5P_!SC1_3P3 (I/O), BC40D_H_PU_ON_5P_SC1_3P3 (I/O), BC40D_H_PUPDOFF_10P_SC1_1P8 (I/O), BC40D_H_PD_ON_10P_!SC1_1P8 (I/O), BC40D_H_PD_ON_10P_SC1_1P8 (I/O), BC40D_H_PU_ON_10P_!SC1_1P8 (I/O), BC40D_H_PUPDOFF_10P_!SC1_1P8 (I/O), BC40D_H_PU_ON_10P_SC1_1P8 (I/O), BC40D_H_PUPDOFF_10P_SC1_3P3 (I/O), BC40D_H_PD_ON_10P_!SC1_3P3 (I/O), BC40D_H_PD_ON_10P_SC1_3P3 (I/O), BC40D_H_PU_ON_10P_!SC1_3P3 (I/O), BC40D_H_PUPDOFF_10P_!SC1_3P3 (I/O), BC40D_H_PU_ON_10P_SC1_3P3 (I/O), BC40D_V_PUPDOFF_5P_SC1_1P8 (I/O), BC40D_V_PD_ON_5P_!SC1_1P8 (I/O), BC40D_V_PD_ON_5P_SC1_1P8 (I/O), BC40D_V_PU_ON_5P_!SC1_1P8 (I/O), BC40D_V_PUPDOFF_5P_!SC1_1P8 (I/O), BC40D_V_PU_ON_5P_SC1_1P8 (I/O), BC40D_V_PUPDOFF_5P_SC1_3P3 (I/O), BC40D_V_PD_ON_5P_!SC1_3P3 (I/O), BC40D_V_PD_ON_5P_SC1_3P3 (I/O), BC40D_V_PU_ON_5P_!SC1_3P3 (I/O), BC40D_V_PUPDOFF_5P_!SC1_3P3 (I/O), BC40D_V_PU_ON_5P_SC1_3P3 (I/O), BC40D_V_PUPDOFF_10P_SC1_1P8 (I/O), BC40D_V_PD_ON_10P_!SC1_1P8 (I/O), BC40D_V_PD_ON_10P_SC1_1P8 (I/O), BC40D_V_PU_ON_10P_!SC1_1P8 (I/O), BC40D_V_PUPDOFF_10P_!SC1_1P8 (I/O), BC40D_V_PU_ON_10P_SC1_1P8 (I/O), BC40D_V_PUPDOFF_10P_SC1_3P3 (I/O), BC40D_V_PD_ON_10P_!SC1_3P3 (I/O), BC40D_V_PD_ON_10P_SC1_3P3 (I/O), BC40D_V_PU_ON_10P_!SC1_3P3 (I/O), BC40D_V_PUPDOFF_10P_!SC1_3P3 (I/O), BC40D_V_PU_ON_10P_SC1_3P3 (I/O), BI2C1833_NORAML_5P_1P8 (I/O_open_drain), BI2C1833_NORAML_5P_3P3 (I/O_open_drain), BI2C1833_NORAML_10P_1P8 (I/O_open_drain), BI2C1833_NORAML_10P_3P3 (I/O_open_drain), IHHV_NORAML_5P_1P8 (Input), IHHV_NORAML_5P_3P3 (Input), IHHV_NORAML_10P_1P8 (Input), IHHV_NORAML_10P_3P3 (Input), IQ_SSDHH_PD_ON_5P_1P8 (Input), IQ_SSDHH_PU_ON_5P_1P8 (Input), IQ_SSDHH_PUPDOFF_5P_1P8 (Input), IQ_SSDHH_PD_ON_5P_3P3 (Input), IQ_SSDHH_PU_ON_5P_3P3 (Input), IQ_SSDHH_PUPDOFF_5P_3P3 (Input), IQ_SSDHH_PD_ON_10P_1P8 (Input), IQ_SSDHH_PU_ON_10P_1P8 (Input), IQ_SSDHH_PUPDOFF_10P_1P8 (Input), IQ_SSDHH_PD_ON_10P_3P3 (Input), IQ_SSDHH_PU_ON_10P_3P3 (Input), IQ_SSDHH_PUPDOFF_10P_3P3 (Input)
